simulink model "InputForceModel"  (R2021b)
settings: Solver=FixedStepAuto  StartTime=0  StopTime=endTime  FixedStep=Ts  RelTol=1e-3
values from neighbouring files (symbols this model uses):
  a = 0.27    [CompareGazeboSimulink.m]    (also in RobotModel.m)
  b = 0.31    [CompareGazeboSimulink.m]    (also in RobotModel.m)
  fro = 0.02    [CompareGazeboSimulink.m]    (also in RobotModel.m)
  fsl = 0.8    [CompareGazeboSimulink.m]    (also in RobotModel.m)
  fsly = 0.8    [CompareGazeboSimulink.m]    (also in RobotModel.m)
  I = (1/12)*m*((2*t)^2 + 0.12^2) + 1.5    (= 2.384)    [CompareGazeboSimulink.m]    (also in RobotModel.m = 0.866666666667)
  ko = 0    [CompareGazeboSimulink.m]    (also in RobotModel.m = 0.25)
  kt = 0.58    [CompareGazeboSimulink.m]    (also in RobotModel.m)
  m = 51    [CompareGazeboSimulink.m]    (also in RobotModel.m = 50)
  mdy = 10    [CompareGazeboSimulink.m]    (also in RobotModel.m)
  momentL = 40    [CompareGazeboSimulink.m]
  momentR = 100    [CompareGazeboSimulink.m]
  mst = 10    [CompareGazeboSimulink.m]    (also in RobotModel.m)
  r = 0.19    [CompareGazeboSimulink.m]    (also in RobotModel.m)
  startStepTime = 2    [CompareGazeboSimulink.m]
  Th0 = 0    [CompareGazeboSimulink.m]    (also in RobotModel.m = 0.9714)
  Th_vel0 = 0    [CompareGazeboSimulink.m]    (also in RobotModel.m)
  X0 = 0    [CompareGazeboSimulink.m]    (also in RobotModel.m)
  x_vel0 = 0    [CompareGazeboSimulink.m]    (also in RobotModel.m)
  Y0 = 0    [CompareGazeboSimulink.m]    (also in RobotModel.m = 2.5)

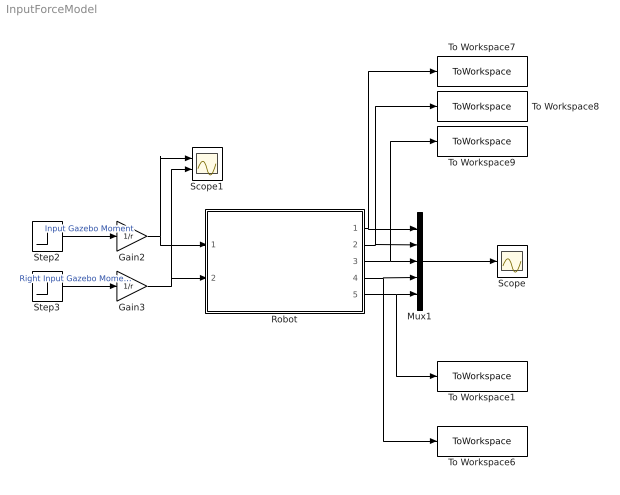
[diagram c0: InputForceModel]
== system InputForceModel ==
  Gain2 : Gain  Gain=1/r
  Gain3 : Gain  Gain=1/r
  Mux1 : Mux  Inputs=5
  Robot : Subsystem
  Scope : Scope
  Scope1 : Scope  NumInputPorts=2
  Step2 : Step  Time=startStepTime  After=momentL  SampleTime=0
  Step3 : Step  Time=startStepTime  After=momentR  SampleTime=0
  To Workspace1 : ToWorkspace  VariableName=simLinearX  SaveFormat=Timeseries  SampleTime=-1
  To Workspace6 : ToWorkspace  VariableName=simAngular  SaveFormat=Timeseries  SampleTime=-1
  To Workspace7 : ToWorkspace  VariableName=simX  SaveFormat=Timeseries  SampleTime=-1
  To Workspace8 : ToWorkspace  VariableName=simY  SaveFormat=Timeseries  SampleTime=-1
  To Workspace9 : ToWorkspace  VariableName=simTheta  SaveFormat=Timeseries  SampleTime=-1
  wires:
  Robot/4(Theta') -> To Workspace6/1, Mux1/4
  Robot/5(v) -> To Workspace1/1, Mux1/5
  Robot/2(Y) -> To Workspace8/1, Mux1/2
  Robot/1(X) -> To Workspace7/1, Mux1/1
  Robot/3(Theta) -> To Workspace9/1, Mux1/3
  Gain2/1 -> Scope1/1, Robot/1(Left Force)
  Gain3/1 -> Scope1/2, Robot/2(Right Force)
  Mux1/1 -> Scope/1
  Step2/1 -> Gain2/1  "Input Gazebo Moment"
  Step3/1 -> Gain3/1  "Right Input Gazebo Moment"

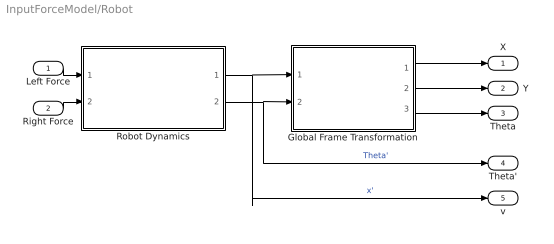
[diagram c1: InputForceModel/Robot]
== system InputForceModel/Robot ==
  Left Force : Inport
  Right Force : Inport  Port=2
  Global Frame Transformation : Subsystem
  Robot Dynamics : Subsystem
  X : Outport
  Y : Outport  Port=2
  Theta : Outport  Port=3
  Theta' : Outport  Port=4
  v : Outport  Port=5
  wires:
  Right Force/1 -> Robot Dynamics/2(Right Force)
  Global Frame Transformation/1(X) -> X/1
  Robot Dynamics/1(x') -> v/1, Global Frame Transformation/1(x')  "x'"
  Left Force/1 -> Robot Dynamics/1(Left Force)
  Robot Dynamics/2(Theta') -> Theta'/1, Global Frame Transformation/2(Theta')  "Theta'"
  Global Frame Transformation/3(Theta) -> Theta/1
  Global Frame Transformation/2(Y) -> Y/1

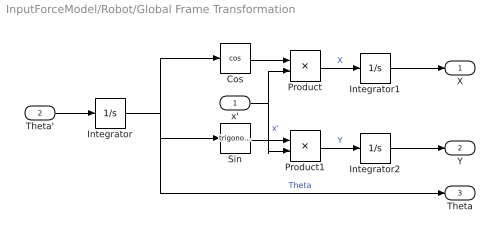
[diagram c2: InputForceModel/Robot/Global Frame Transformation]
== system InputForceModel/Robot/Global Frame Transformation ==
  x' : Inport
  Theta' : Inport  Port=2
  Cos : Trigonometry  Operator=cos
  Integrator : Integrator  InitialCondition=Th0
  Integrator1 : Integrator  InitialCondition=X0
  Integrator2 : Integrator  InitialCondition=Y0
  Product : Product
  Product1 : Product
  Sin : Trigonometry
  X : Outport
  Y : Outport  Port=2
  Theta : Outport  Port=3
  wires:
  Product1/1 -> Integrator2/1  "Y"
  Integrator/1 -> Theta/1, Sin/1, Cos/1  "Theta"
  x'/1 -> Product1/2, Product/2  "x'"
  Sin/1 -> Product1/1
  Cos/1 -> Product/1
  Product/1 -> Integrator1/1  "X"
  Theta'/1 -> Integrator/1
  Integrator1/1 -> X/1
  Integrator2/1 -> Y/1

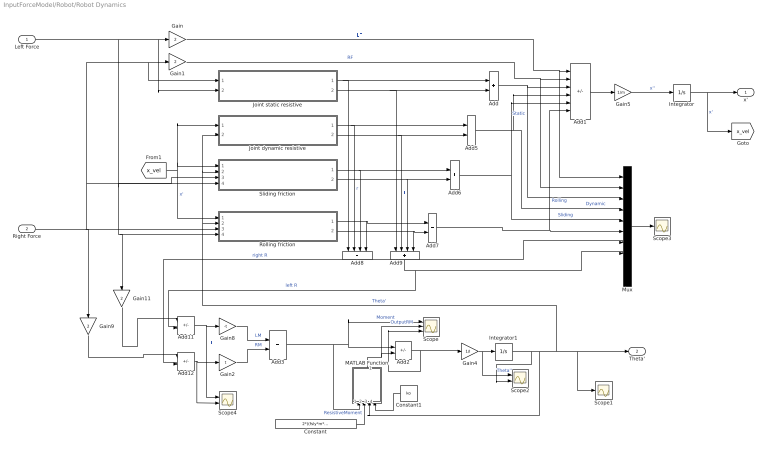
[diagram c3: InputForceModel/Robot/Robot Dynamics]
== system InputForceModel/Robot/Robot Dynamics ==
  Left Force : Inport
  Right Force : Inport  Port=2
  Add{,3,5..7} (5 alike) : Sum
  Add1 : Sum  Inputs=++----
  Add11 : Sum  Inputs=+-
  Add12 : Sum  Inputs=+-
  Add2 : Sum  Inputs=+-
  Add8 : Sum  Inputs=++++
  Add9 : Sum  Inputs=++++
  Constant : Constant  Value=2*((fsly*m*9.81)/(a+b))*a*b*kt
  Constant1 : Constant  Value=ko
  Gain{,1,9,11} (4 alike) : Gain  Gain=2
  Gain2 : Gain  Gain=t
  Gain4 : Gain  Gain=1/I
  Gain5 : Gain  Gain=1/m
  Gain8 : Gain  Gain=-t
  Integrator : Integrator  InitialCondition=x_vel0
  Integrator1 : Integrator  InitialCondition=Th_vel0
  Joint dynamic resistive : Subsystem
  Joint static resistive : Subsystem
  MATLAB Function : MATLAB Function  TreatAsAtomicUnit=on
  Mux : Mux  Inputs=10
  Rolling friction : Subsystem
  Scope : Scope  NumInputPorts=3
  Scope1 : Scope
  Scope2 : Scope  NumInputPorts=2
  Scope3 : Scope
  Scope4 : Scope  NumInputPorts=2
  Sliding friction : Subsystem
  x' : Outport
  Theta' : Outport  Port=2
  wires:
  Gain4/1 -> Scope2/1, Integrator1/1  "Theta''"
  Integrator1/1 -> Scope2/2, Sliding friction/2(Theta'), Joint dynamic resistive/2(Theta'), Rolling friction/2(Theta'), Scope1/1, Theta'/1, MATLAB Function/3(Omega)  "Theta'"
  Gain1/1 -> Mux/2, Add1/2  "RF"
  Add1/1 -> Gain5/1
  Gain5/1 -> Integrator/1  "x''"
  Integrator/1 -> x'/1, [x_vel]  "x'"
  [x_vel] -> Joint dynamic resistive/1("Local Long Velocity "), Sliding friction/1(Local longitudal velocity), Rolling friction/1(Local longitudal velocity)  "x'"
  Joint static resistive/2(Static Resistive Force Left) -> Add9/1, Add/2
  Joint dynamic resistive/1(Dynamic Resistive Force Right) -> Add8/2, Add5/1  "r"
  Joint dynamic resistive/2(Dynamic Resistive Force Left) -> Add9/2, Add5/2  "l"
  Sliding friction/1(Friction Right Force) -> Add8/3, Add6/1
  Sliding friction/2(Friction Left Force) -> Add9/3, Add6/2
  Rolling friction/1(Friction Right Force) -> Add8/4, Add7/1
  Rolling friction/2(Friction Left Force) -> Add9/4, Add7/2
  Add/1 -> Add1/3, Mux/3  "Static"
  Add6/1 -> Add1/5, Mux/5  "Sliding"
  Add7/1 -> Mux/6, Add1/6  "Rolling"
  Add5/1 -> Mux/4, Add1/4  "Dynamic"
  Add9/1 -> Add11/2, Mux/8  "left R"
  Add8/1 -> Add12/2, Mux/7  "right R"
  Mux/1 -> Scope3/1
  Add11/1 -> Scope4/1, Gain8/1  "LL"
  Add12/1 -> Scope4/2, Gain2/1
  Gain9/1 -> Add12/1
  Gain11/1 -> Add11/1
  Gain8/1 -> Add3/1  "LM"
  Gain2/1 -> Add3/2  "RM"
  Gain/1 -> Mux/1, Add1/1  "LF"
  Joint static resistive/1(Static Resistive Force Right) -> Add8/1, Add/1
  Add2/1 -> Scope/3, Gain4/1
  Add3/1 -> Scope/1, Add2/1, MATLAB Function/1(Moment)  "Moment"
  MATLAB Function/1(y) -> Scope/2, Add2/2  "OutputRM"
  Constant/1 -> MATLAB Function/2(ResistiveMoment)  "ResistiveMoment"
  Left Force/1 -> Gain11/1, Rolling friction/4(Fl), Sliding friction/4(Fl), Joint static resistive/2("Fl "), Gain/1
  Right Force/1 -> Gain9/1, Rolling friction/3(Fr), Sliding friction/3(Fr), Joint static resistive/1(Fr), Gain1/1
  Constant1/1 -> MATLAB Function/4(ko)

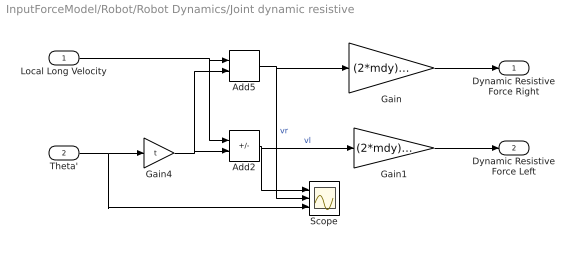
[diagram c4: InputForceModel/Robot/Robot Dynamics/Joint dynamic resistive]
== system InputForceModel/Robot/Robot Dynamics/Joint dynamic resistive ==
  "Local Long Velocity " : Inport
  Theta' : Inport  Port=2
  Add2 : Sum  Inputs=+-
  Add5 : Sum
  Gain : Gain  Gain=(2*mdy)/(r*r)
  Gain1 : Gain  Gain=(2*mdy)/(r*r)
  Gain4 : Gain  Gain=t
  Scope : Scope  NumInputPorts=3
  Dynamic Resistive Force Right : Outport
  Dynamic Resistive Force Left : Outport  Port=2
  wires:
  Gain/1 -> Dynamic Resistive Force Right/1
  Gain1/1 -> Dynamic Resistive Force Left/1
  Gain4/1 -> Add5/2, Add2/2
  Theta'/1 -> Scope/3, Gain4/1
  Add5/1 -> Scope/2, Gain/1  "vr"
  Add2/1 -> Scope/1, Gain1/1  "vl"
  "Local Long Velocity "/1 -> Add2/1, Add5/1

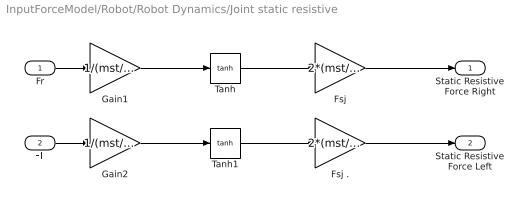
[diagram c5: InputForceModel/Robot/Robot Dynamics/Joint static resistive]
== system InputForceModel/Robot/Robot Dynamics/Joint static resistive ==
  Fr : Inport
  "Fl " : Inport  Port=2
  Fsj : Gain  Gain=2*(mst/r)
  Fsj . : Gain  Gain=2*(mst/r)
  Gain1 : Gain  Gain=1/(mst/r)
  Gain2 : Gain  Gain=1/(mst/r)
  Tanh : Trigonometry  Operator=tanh
  Tanh1 : Trigonometry  Operator=tanh
  Static Resistive Force Right : Outport
  Static Resistive Force Left : Outport  Port=2
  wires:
  Fr/1 -> Gain1/1
  "Fl "/1 -> Gain2/1
  Tanh/1 -> Fsj/1
  Tanh1/1 -> Fsj ./1
  Gain1/1 -> Tanh/1
  Gain2/1 -> Tanh1/1
  Fsj/1 -> Static Resistive Force Right/1
  Fsj ./1 -> Static Resistive Force Left/1

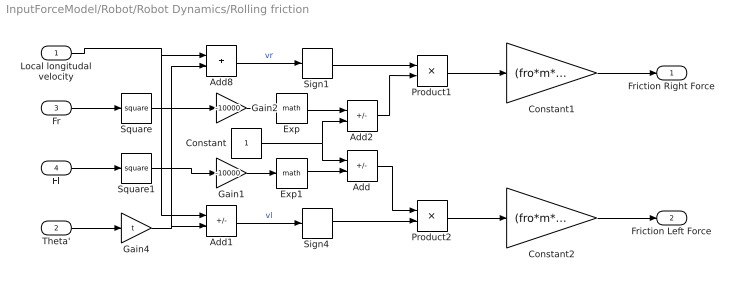
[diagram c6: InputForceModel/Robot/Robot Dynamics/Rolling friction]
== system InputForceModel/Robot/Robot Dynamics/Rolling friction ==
  Local longitudal velocity : Inport
  Theta' : Inport  Port=2
  Fr : Inport  Port=3
  Fl : Inport  Port=4
  Add : Sum  Inputs=+-
  Add1 : Sum  Inputs=+-
  Add2 : Sum  Inputs=-+
  Add8 : Sum
  Constant : Constant
  Constant1 : Gain  Gain=(fro*m*9.81)/2
  Constant2 : Gain  Gain=(fro*m*9.81)/2
  Exp : Math
  Exp1 : Math
  Gain1 : Gain  Gain=-10000
  Gain2 : Gain  Gain=-10000
  Gain4 : Gain  Gain=t
  Product1 : Product
  Product2 : Product
  Sign1 : Signum
  Sign4 : Signum
  Square : Math  Operator=square
  Square1 : Math  Operator=square
  Friction Right Force : Outport
  Friction Left Force : Outport  Port=2
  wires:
  Sign1/1 -> Product1/1
  Sign4/1 -> Product2/2
  Add8/1 -> Sign1/1  "vr"
  Fl/1 -> Square1/1
  Fr/1 -> Square/1
  Square1/1 -> Gain1/1
  Gain4/1 -> Add1/2, Add8/2
  Theta'/1 -> Gain4/1
  Add1/1 -> Sign4/1  "vl"
  Square/1 -> Gain2/1
  Gain2/1 -> Exp/1
  Gain1/1 -> Exp1/1
  Add2/1 -> Product1/2
  Add/1 -> Product2/1
  Exp1/1 -> Add/2
  Exp/1 -> Add2/1
  Constant/1 -> Add2/2, Add/1
  Local longitudal velocity/1 -> Add1/1, Add8/1
  Product1/1 -> Constant1/1
  Product2/1 -> Constant2/1
  Constant2/1 -> Friction Left Force/1
  Constant1/1 -> Friction Right Force/1

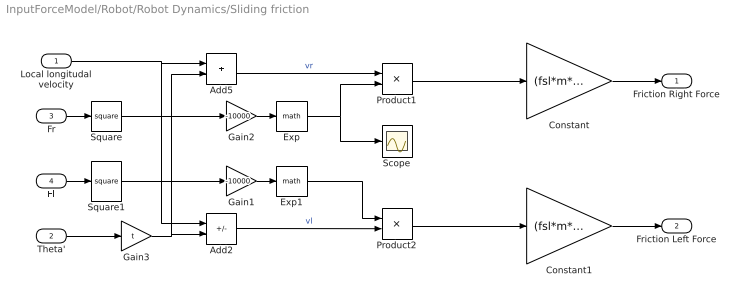
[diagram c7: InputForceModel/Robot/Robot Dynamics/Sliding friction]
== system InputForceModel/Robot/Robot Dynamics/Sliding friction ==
  Local longitudal velocity : Inport
  Theta' : Inport  Port=2
  Fr : Inport  Port=3
  Fl : Inport  Port=4
  Add2 : Sum  Inputs=+-
  Add5 : Sum
  Constant : Gain  Gain=(fsl*m*9.81)/2
  Constant1 : Gain  Gain=(fsl*m*9.81)/2
  Exp : Math
  Exp1 : Math
  Gain1 : Gain  Gain=-10000
  Gain2 : Gain  Gain=-10000
  Gain3 : Gain  Gain=t
  Product1 : Product
  Product2 : Product
  Scope : Scope
  Square : Math  Operator=square
  Square1 : Math  Operator=square
  Friction Right Force : Outport
  Friction Left Force : Outport  Port=2
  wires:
  Theta'/1 -> Gain3/1
  Gain3/1 -> Add2/2, Add5/2
  Add5/1 -> Product1/1  "vr"
  Add2/1 -> Product2/2  "vl"
  Exp/1 -> Scope/1, Product1/2
  Gain1/1 -> Exp1/1
  Gain2/1 -> Exp/1
  Fr/1 -> Square/1
  Fl/1 -> Square1/1
  Square/1 -> Gain2/1
  Square1/1 -> Gain1/1
  Product1/1 -> Constant/1
  Product2/1 -> Constant1/1
  Exp1/1 -> Product2/1
  Local longitudal velocity/1 -> Add2/1, Add5/1
  Constant/1 -> Friction Right Force/1
  Constant1/1 -> Friction Left Force/1

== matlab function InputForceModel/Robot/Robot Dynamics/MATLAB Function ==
function y = fcn(Moment, ResistiveMoment, Omega, ko)
    y = ResistiveMoment;
    
    %if(Omega ~= 0) 
        if(abs(Moment) < abs(ResistiveMoment))
            y = Moment;
        else
            y = (ko*Omega + sign(Omega))*ResistiveMoment;
        end
    %else
        %y = Moment;  % 0


end
